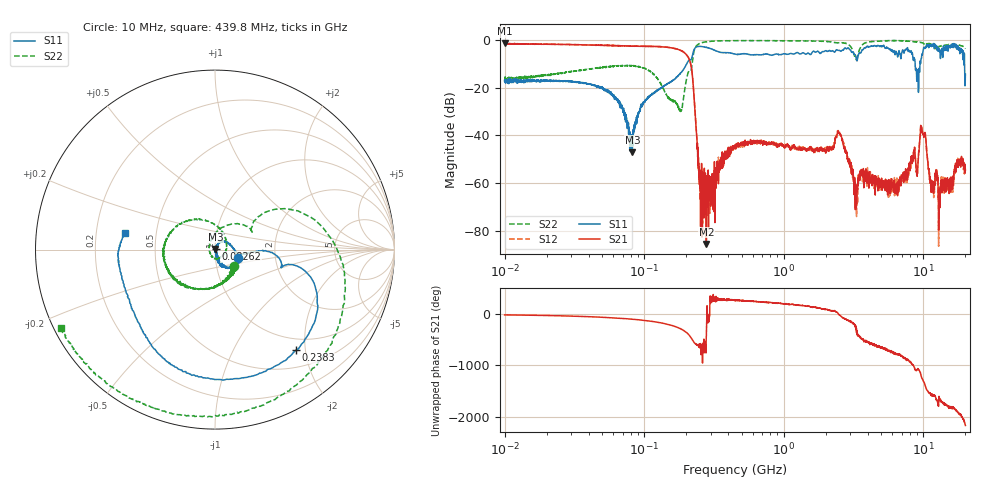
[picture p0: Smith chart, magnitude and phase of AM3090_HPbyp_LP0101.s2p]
# Hz S DB R 50
!freq MagS11 AngS11 MagS21 AngS21 MagS12 AngS12 MagS22 AngS22
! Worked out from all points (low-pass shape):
!   3201 points, 10 MHz to 20 GHz, reference 50 ohm
!   highest |S21| = -1.34 dB at 10.05 MHz (marker M1); lowest = -85.6 dB at 278.8 MHz (marker M2)
!   |S21| within 3 dB of the highest: start of sweep to 181.3 MHz
!   lowest |S11| = -47.2 dB at 82.23 MHz (marker M3), VSWR 1.01, Z = 50.2 + j0.367 ohm
!   |S11| at or under -10 dB: start of sweep to 201.6 MHz; 8.731 GHz to 9.453 GHz (722.1 MHz wide, 7.94 % of centre); 19.73 GHz to end of sweep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
!   |S22| runs from -30.1 to -0.2 dB; largest |S21 - S12| = 0.035
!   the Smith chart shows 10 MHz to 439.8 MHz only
!   S11 on the Smith chart (normalised r, x): 10 MHz: 1.29, -0.12; 82.62 MHz: 1.01, +0.01; 238.3 MHz: 0.78, -1.82; 439.8 MHz: 0.33, +0.08
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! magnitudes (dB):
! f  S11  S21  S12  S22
! 10 MHz  -17.3  -1.6  -1.5  -17.3
! 10.05 MHz  -17.3  -1.3  -1.6  -17.6
! 35.55 MHz  -18.0  -2.1  -2.0  -12.7
! 60.52 MHz  -23.0  -2.4  -2.4  -11.0
! 82.23 MHz  -47.2  -2.6  -2.5  -11.0
! 82.62 MHz  -44.6  -2.6  -2.5  -10.9
! 126.1 MHz  -21.1  -2.8  -2.8  -16.7
! 180.9 MHz  -14.1  -4.3  -4.3  -29.8
! 208.6 MHz  -8.6  -7.7  -7.7  -13.0
! 238.3 MHz  -2.9  -41.7  -41.5  -2.3
! 252.3 MHz  -2.7  -54.6  -57.3  -1.4
! 278.8 MHz  -3.1  -85.6  -73.3  -0.8
! 439.8 MHz  -5.8  -45.5  -44.7  -0.3
! 447.2 MHz  -5.9  -44.7  -44.8  -0.3
! 1.59 GHz  -5.4  -45.6  -45.5  -0.5
! 2.491 GHz  -4.4  -39.1  -38.4  -1.2
! 3.297 GHz  -7.6  -69.6  -64.9  -8.1
! 5.639 GHz  -3.6  -58.5  -62.9  -0.3
! 9.025 GHz  -14.5  -57.2  -54.5  -0.9
! 9.878 GHz  -5.5  -39.4  -38.7  -1.2
! 11.55 GHz  -1.8  -59.1  -62.8  -2.1
! 20 GHz  -14.4  -54.7  -53.4  -3.7
